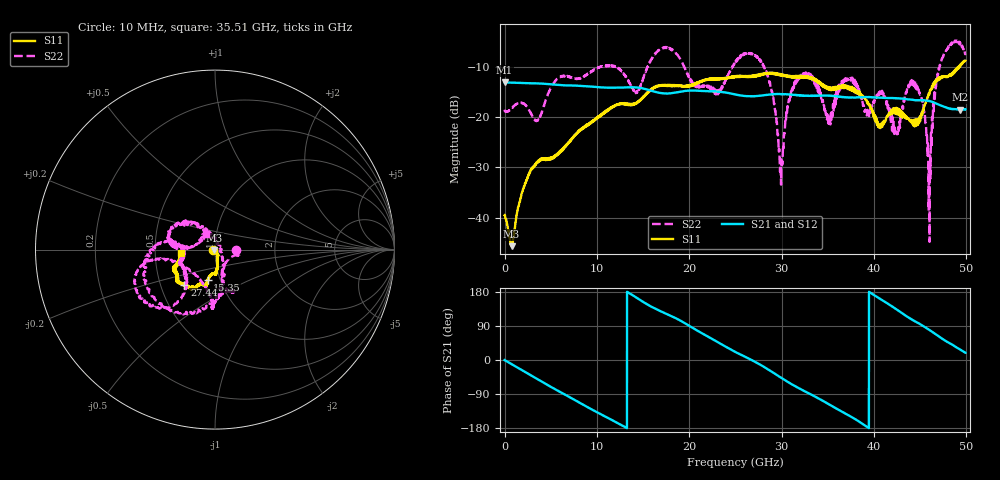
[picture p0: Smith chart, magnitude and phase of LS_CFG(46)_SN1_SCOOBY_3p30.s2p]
!Keysight Technologies,N5245B,MY58422026,A.13.80.08
!Date: Thursday, March 19, 2020 23:41:17
!Correction: S11(Full 2 Port(1,2))
!S21(Full 2 Port(1,2))
!S12(Full 2 Port(1,2))
!S22(Full 2 Port(1,2))
!S2P File: Measurements: S11, S21, S12, S22:
# Hz S DB R 50.0
!freq dBS11 angS11 dBS21 angS21 dBS12 angS12 dBS22 angS22
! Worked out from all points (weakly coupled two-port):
!   4991 points, 10 MHz to 49.91 GHz, reference 50 ohm
!   highest |S21| = -13.06 dB at 10 MHz (marker M1); lowest = -18.5 dB at 49.34 GHz (marker M2)
!   lowest |S11| = -45.7 dB at 760 MHz (marker M3), VSWR 1.01, Z = 49.7 - j0.393 ohm
!   |S11| at or under -10 dB: start of sweep to 49.13 GHz; 49.16206 GHz to 49.22798 GHz (65.92 MHz wide, 0.134 % of centre)
!   |S22| runs from -44.8 to -4.7 dB; largest |S21 - S12| = 0.0021
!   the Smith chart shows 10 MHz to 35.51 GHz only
!   S11 on the Smith chart (normalised r, x): 10 MHz: 0.98, -0.01; 15.35 GHz: 0.87, -0.30; 27.44 GHz: 0.66, -0.28; 35.51 GHz: 0.68, -0.03
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1e7  -39.49 -165.1  -13.06 -0.3  -13.05 -0.3  -18.50 0.1
7.6e8  -45.69 -130.5  -13.11 -10.9  -13.10 -10.9  -18.25 -13.2
2.87e9  -30.50 -56.7  -13.23 -40.4  -13.22 -40.4  -19.27 -18.7
8.33e9  -22.50 -80.2  -13.74 -115.5  -13.74 -115.4  -12.13 -79.3
1.535e10  -15.28 -103.9  -14.45 148.2  -14.44 148.3  -10.50 -169.8
1.665e10  -13.80 -104.0  -15.08 131.5  -15.07 131.5  -6.74 -162.3
2.299e10  -12.43 -116.9  -14.86 48.7  -14.87 48.8  -15.32 -171.9
2.496e10  -11.98 -122.5  -15.42 21.7  -15.41 21.9  -9.24 -179.4
2.744e10  -11.68 -130.8  -15.74 -8.9  -15.74 -8.8  -8.23 -114.8
2.893e10  -11.35 -140.3  -15.44 -30.8  -15.43 -30.5  -14.91 -76.4
2.991e10  -11.54 -143.3  -15.42 -46.3  -15.42 -46.1  -31.63 14.9
3.116e10  -11.88 -147.1  -15.51 -64.7  -15.52 -64.4  -14.28 133.6
3.328e10  -12.21 -158.1  -15.72 -92.3  -15.72 -91.9  -12.04 172.9
3.551e10  -14.39 -174.5  -15.72 -122.4  -15.66 -121.9  -19.83 119.1
3.734e10  -14.41 172.7  -16.06 -147.3  -15.97 -147.4  -12.43 137.0
4.16e10  -19.27 105.5  -16.17 147.2  -16.19 147.1  -18.40 26.7
4.249e10  -19.43 102.0  -16.22 132.9  -16.25 132.8  -23.18 -11.4
4.445e10  -21.00 53.6  -16.60 102.1  -16.61 102.3  -13.06 -19.3
4.601e10  -15.39 6.9  -16.75 79.3  -16.77 79.4  -35.76 -16.3
4.711e10  -12.03 9.4  -17.55 61.0  -17.56 61.1  -9.80 -98.9
4.934e10  -9.81 -16.8  -18.47 27.6  -18.48 27.7  -5.08 -34.5
4.991e10  -8.72 -14.6  -18.41 19.3  -18.43 19.2  -7.36 -21.1
